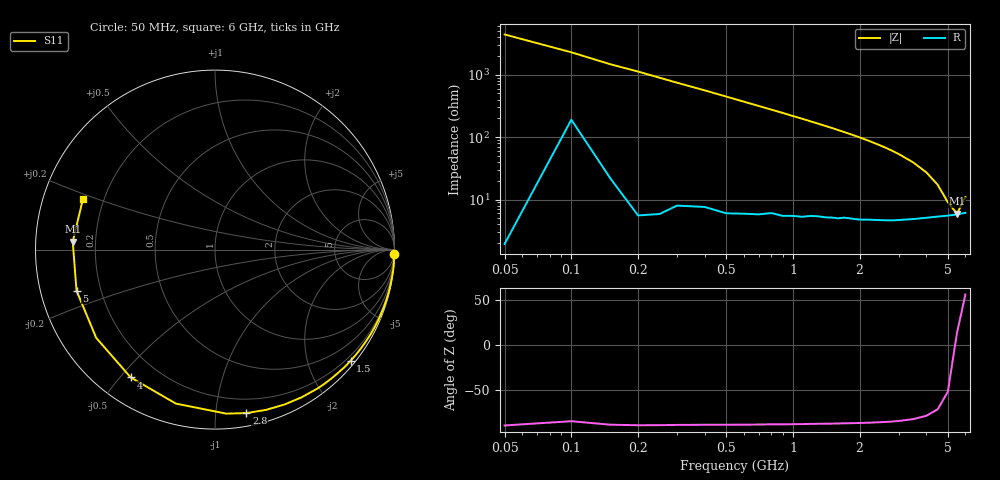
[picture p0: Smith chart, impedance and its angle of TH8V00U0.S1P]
! SIEMENS Discrete & RF Semiconductors
! BAS70
! Si Schottky Diode in SOT23
! VR = 8 V
! S-Parameters:  February  1997
# GHz  S  MA  R  50
!  f  S11
! GHz  MAG  ANG
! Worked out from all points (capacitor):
!   34 points, 50 MHz to 6 GHz, reference 50 ohm
!   read as one part to ground: C = 722 fF near 50 MHz
!   lowest |Z| = 5.92 ohm at 5.5 GHz (marker M1)
!   series resonance near 5.419 GHz, so ESL is about 1.2 nH
!   S11 on the Smith chart (normalised r, x): 50 MHz: 0, -88; 1.5 GHz: 0.10, -2.80; 2.8 GHz: 0.09, -1.21; 4 GHz: 0.10, -0.53; 5 GHz: 0.11, -0.14; 6 GHz: 0.12, +0.18
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0.05  1 -1.3
0.1  0.9964 -2.5
0.15  0.999 -3.9
0.2  0.9996 -5.1
0.4  0.9976 -10.2
0.5  0.997 -12.8
0.6  0.9958 -15.4
0.7  0.9943 -18.0
0.8  0.9923 -20.6
0.9  0.9912 -23.2
1  0.9891 -25.9
1.1  0.9873 -28.5
1.3  0.9819 -33.9
1.5  0.977 -39.3
1.6  0.9744 -42.2
1.8  0.9677 -47.8
2  0.9619 -53.6
2.2  0.9539 -59.7
2.4  0.9459 -65.9
2.6  0.9372 -72.3
2.8  0.9275 -79.1
3  0.9162 -86.0
3.5  0.8854 -104.2
4  0.8531 -123.4
4.5  0.8245 -143.4
5  0.8047 -163.5
5.5  0.7937 176.8
6  0.7879 159.1
